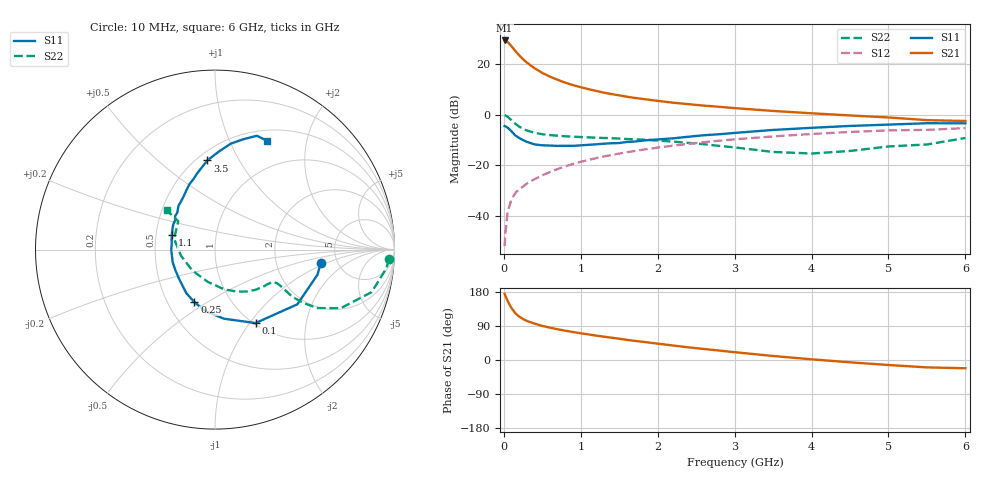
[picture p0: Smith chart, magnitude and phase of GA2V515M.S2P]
! Infineon Technologies  Discrete & RF Semiconductors
! BF775
! Si NPN RF Bipolar Junction Transistor in SOT23
! VCE = 2.5 V  IC = 15 mA
! Common Emitter S-Parameters:  May  1996
# GHz  S  MA  R  50
!  f  S11  S21  S12  S22
! GHz  MAG  ANG  MAG  ANG  MAG  ANG  MAG  ANG
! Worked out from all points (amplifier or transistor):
!   36 points, 10 MHz to 6 GHz, reference 50 ohm
!   highest |S21| = 29.1 dB at 10 MHz (marker M1)
!   |S21| within 3 dB of that: start of sweep to 118.9 MHz
!   unconditionally stable (mu >= 1): 431 MHz to 3.41 GHz
!   at 250 MHz: K = 0.81, MSG = 25.0 dB, |S12| = -28.2 dB
!   at 1.4 GHz: K = 1.12, MAG = 9.9 dB, |S12| = -15.9 dB
!   at 6 GHz: K = 0.97, MSG = 1.4 dB, |S12| = -5.3 dB
!   S11 on the Smith chart (normalised r, x): 10 MHz: 3.73, -0.85; 100 MHz: 1.02, -1.07; 250 MHz: 0.68, -0.44; 1.1 GHz: 0.60, +0.11; 3.5 GHz: 0.56, +0.75; 6 GHz: 0.63, +1.39
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0.01  0.5948 -7.1  28.54 174.8  0.0026 87.3  0.9725 -3.1
0.02  0.5877 -13.8  28.33 169.3  0.0047 79.6  0.9592 -6.4
0.05  0.5508 -33.6  26.59 155.3  0.0125 76.0  0.9042 -15.2
0.1  0.4675 -61.1  21.91 136.7  0.0217 67.7  0.7726 -25.0
0.15  0.3882 -82.6  17.69 123.2  0.0288 64.2  0.6596 -29.6
0.2  0.3468 -98.9  14.56 114.5  0.0341 64.5  0.5793 -31.1
0.25  0.3144 -111.4  12.19 108.0  0.0388 63.6  0.5237 -31.3
0.3  0.2909 -123.2  10.47 103.1  0.0441 64.7  0.4864 -31.0
0.4  0.2592 -140.0  8.112 95.9  0.0539 66.2  0.4386 -29.6
0.5  0.249 -152.2  6.57 90.0  0.0639 67.2  0.4107 -28.8
0.6  0.2461 -163.5  5.557 85.3  0.0747 67.6  0.3952 -28.5
0.7  0.2423 -173.3  4.813 81.1  0.085 67.7  0.384 -28.7
0.8  0.2438 -179.9  4.228 77.3  0.0963 67.4  0.3741 -29.0
0.9  0.2431 172.6  3.786 73.8  0.1071 67.0  0.3674 -29.5
1.1  0.2544 161.3  3.154 67.5  0.1284 65.8  0.3566 -32.0
1.3  0.2677 151.8  2.696 61.6  0.1502 64.1  0.3467 -34.5
1.6  0.2901 139.8  2.238 53.1  0.182 61.1  0.3311 -39.7
2.2  0.3414 121.2  1.71 38.2  0.2451 54.4  0.2945 -52.3
3.5  0.4987 94.9  1.178 10.6  0.3719 37.4  0.1843 -102.6
4.5  0.5977 81.4  0.961 -6.1  0.4549 23.9  0.1928 -170.0
5.5  0.6756 69.8  0.777 -19.5  0.5004 9.3  0.2583 142.4
6  0.6724 64.6  0.747 -21.8  0.5425 5.1  0.3465 140.8
